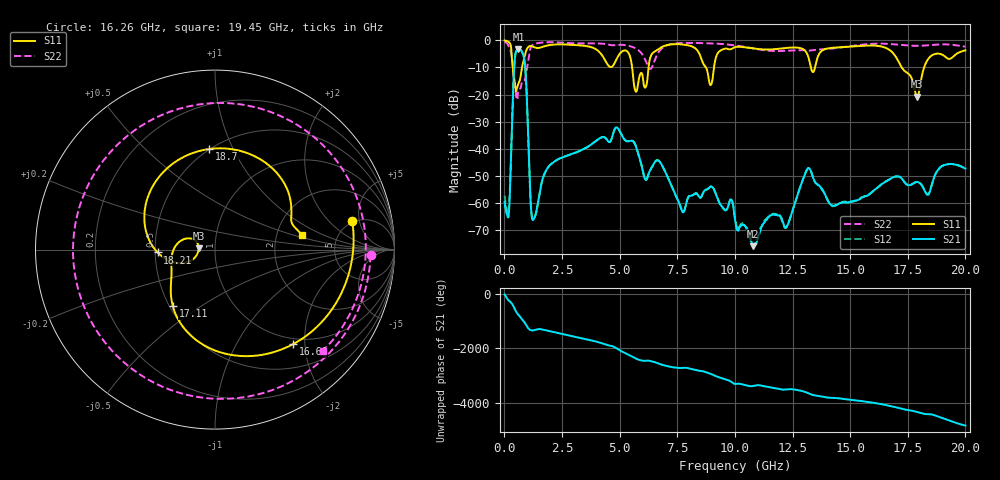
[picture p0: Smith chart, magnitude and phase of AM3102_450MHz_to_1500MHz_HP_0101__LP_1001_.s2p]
!Agilent Technologies,E8364B,MY43040894,A.07.50.67
!Agilent E8364B: A.07.50.67
!Date: Thursday, January 11, 2018 05:42:07
!Correction: S11(Full 2 Port(1,2))
!S21(Full 2 Port(1,2))
!S12(Full 2 Port(1,2))
!S22(Full 2 Port(1,2))
!S2P File: Measurements: S11, S21, S12, S22:
# Hz S  dB  R 50
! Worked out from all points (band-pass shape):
!   1601 points, 10 MHz to 20 GHz, reference 50 ohm
!   highest |S21| = -3.26 dB at 609.7 MHz (marker M1); lowest = -75.9 dB at 10.79 GHz (marker M2)
!   |S21| within 3 dB of the highest: 460.8 MHz to 841.2 MHz (380.4 MHz wide, 58.4 % of centre)
!   lowest |S11| = -20.8 dB at 17.9 GHz (marker M3), VSWR 1.20, Z = 41.7 + j0.643 ohm
!   |S11| at or under -10 dB: 365.6 MHz to 764.4 MHz (398.9 MHz wide, 70.6 % of centre); 5.542 GHz to 6.253 GHz (711.2 MHz wide, 12.1 % of centre); 17.24 GHz to 18.21 GHz (971.9 MHz wide, 5.48 % of centre)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
!   |S22| runs from -21.9 to -0.5 dB; largest |S21 - S12| = 0.0021
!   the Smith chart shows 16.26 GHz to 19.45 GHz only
!   S11 on the Smith chart (normalised r, x): 16.26 GHz: 4.77, +3.97; 16.66 GHz: 0.89, -1.76; 17.11 GHz: 0.52, -0.39; 18.21 GHz: 0.52, -0.02; 18.7 GHz: 0.50, +0.81; 19.45 GHz: 2.78, +0.60
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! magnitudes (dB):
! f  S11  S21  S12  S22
! 10 MHz  -0.1  -59.5  -57.2  -0.5
! 184.9 MHz  -0.6  -64.8  -63.0  -2.2
! 434.8 MHz  -14.8  -8.8  -8.8  -15.3
! 609.7 MHz  -15.9  -3.3  -3.3  -18.5
! 884.6 MHz  -5.7  -8.5  -8.5  -14.6
! 1.259 GHz  -2.4  -66.0  -65.8  -1.6
! 3.346 GHz  -1.9  -40.5  -40.5  -1.2
! 5.707 GHz  -18.9  -39.1  -39.1  -3.0
! 6.682 GHz  -3.3  -44.3  -44.3  -4.5
! 8.943 GHz  -16.5  -54.0  -53.9  -1.1
! 10.01 GHz  -2.5  -65.9  -65.6  -1.9
! 10.79 GHz  -3.0  -75.9  -75.4  -3.0
! 13.34 GHz  -11.3  -49.3  -49.3  -3.7
! 16.26 GHz  -2.1  -53.7  -53.8  -1.2
! 16.66 GHz  -3.3  -51.4  -51.4  -1.3
! 16.68 GHz  -3.4  -51.4  -51.4  -1.3
! 17.11 GHz  -8.1  -50.2  -50.3  -1.7
! 17.9 GHz  -20.8  -52.2  -52.2  -2.0
! 18.21 GHz  -9.9  -55.1  -54.9  -1.9
! 18.7 GHz  -5.0  -49.3  -49.3  -1.6
! 19.45 GHz  -6.2  -45.6  -45.6  -1.7
! 20 GHz  -3.7  -47.2  -47.1  -2.3
